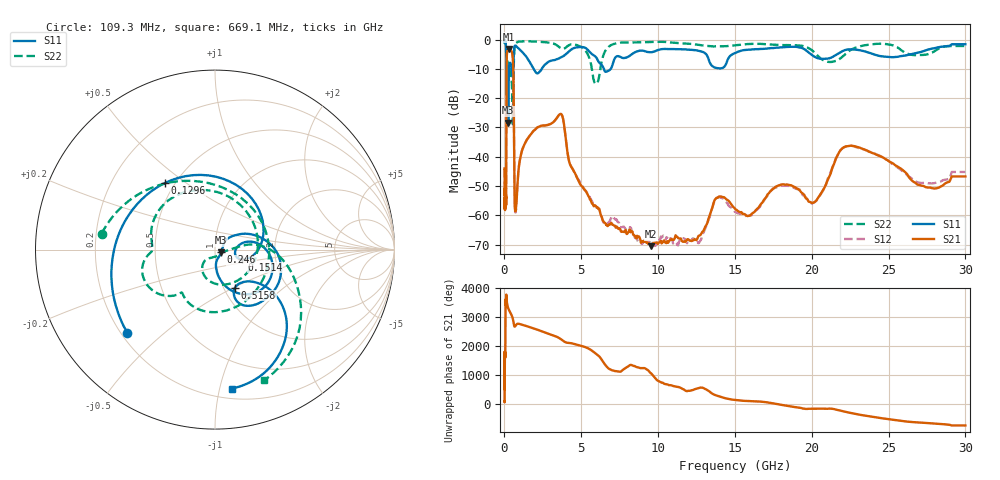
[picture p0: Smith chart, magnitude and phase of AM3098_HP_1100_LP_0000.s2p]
! Date/Time: Thu, Feb 28, 2019 8:43 AM
! Network Analyzer: Agilent Technologies E8364B Rev: A.07.50.67
! Sweep from 0.010 to 30.000 GHz, 1601 Points, Sweep Type: LOG
! Power Supply: 5.022 V, 0.002 A
# Hz S DB R 50
!freq MagS11 AngS11 MagS21 AngS21 MagS12 AngS12 MagS22 AngS22
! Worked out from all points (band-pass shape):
!   1601 points, 10 MHz to 30 GHz, reference 50 ohm
!   highest |S21| = -3.26 dB at 266.5 MHz (marker M1); lowest = -70.6 dB at 9.538 GHz (marker M2)
!   |S21| within 3 dB of the highest: 148.5 MHz to 538.4 MHz (389.8 MHz wide, 114 % of centre)
!   lowest |S11| = -28.4 dB at 246 MHz (marker M3), VSWR 1.08, Z = 53.6 - j1.66 ohm
!   |S11| at or under -10 dB: 204.5 MHz to 302.2 MHz (97.69 MHz wide, 38.6 % of centre); 1.888 GHz to 2.428 GHz (539.7 MHz wide, 25 % of centre); 6.472 GHz to 6.92 GHz (447.7 MHz wide, 6.69 % of centre)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
!   |S22| runs from -28.9 to -0.5 dB; largest |S21 - S12| = 0.01
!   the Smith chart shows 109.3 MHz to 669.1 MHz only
!   S11 on the Smith chart (normalised r, x): 109.3 MHz: 0.22, -0.38; 129.6 MHz: 0.44, +0.42; 151.4 MHz: 1.34, -0.15; 246 MHz: 1.07, -0.03; 515.8 MHz: 1.13, -0.51; 669.1 MHz: 0.28, -1.09
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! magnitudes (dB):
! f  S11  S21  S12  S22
! 10 MHz  -0.4  -44.0  -44.2  -0.5
! 38.04 MHz  -0.4  -57.1  -55.9  -0.6
! 109.3 MHz  -3.4  -52.4  -55.1  -3.9
! 129.6 MHz  -6.7  -21.4  -21.3  -10.3
! 144.7 MHz  -11.8  -7.4  -7.4  -9.3
! 151.4 MHz  -16.0  -5.7  -5.6  -10.2
! 202.3 MHz  -9.7  -3.8  -3.8  -7.5
! 246 MHz  -28.4  -3.3  -3.2  -9.1
! 266.5 MHz  -16.9  -3.3  -3.2  -9.0
! 462 MHz  -9.2  -4.1  -4.1  -13.7
! 515.8 MHz  -12.4  -5.1  -5.1  -25.4
! 550.5 MHz  -11.4  -7.2  -7.2  -27.4
! 593.4 MHz  -5.8  -15.9  -15.9  -12.0
! 669.1 MHz  -2.2  -56.3  -56.3  -2.2
! 2.084 GHz  -11.5  -30.3  -30.3  -0.7
! 3.686 GHz  -6.1  -25.4  -25.4  -3.0
! 5.959 GHz  -6.0  -56.9  -57.1  -15.2
! 7.926 GHz  -6.2  -66.1  -65.3  -1.0
! 9.538 GHz  -4.4  -70.6  -68.6  -0.9
! 20.1 GHz  -5.6  -55.7  -55.7  -4.1
! 22.67 GHz  -3.4  -36.3  -36.4  -3.2
! 30 GHz  -1.6  -46.7  -45.2  -2.2
